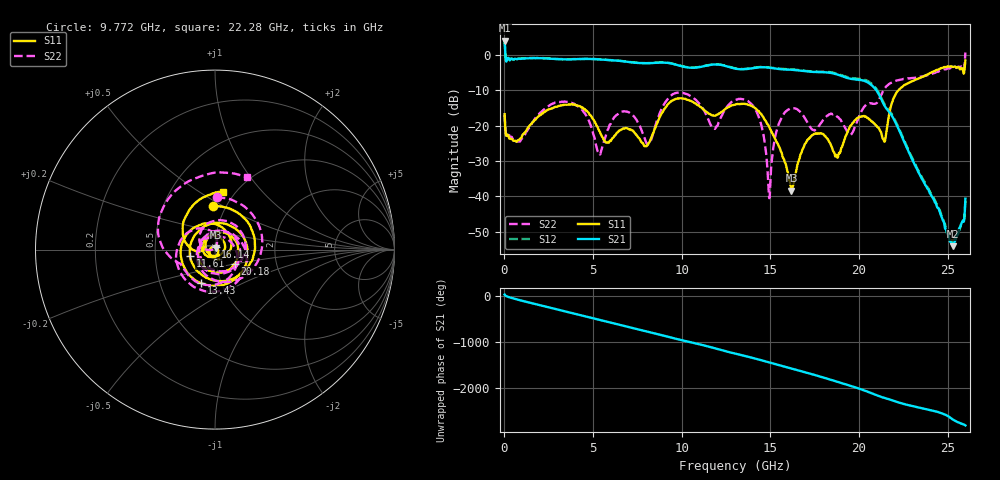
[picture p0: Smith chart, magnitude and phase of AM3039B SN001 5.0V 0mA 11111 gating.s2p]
!Agilent Technologies,E8364B,MY43040894,A.07.50.67
!Agilent E8364B: A.07.50.67
!Date: Tuesday, June 28, 2016 08:13:28
!Correction: S11(Full 2 Port(1,2))
!S21(Full 2 Port(1,2))
!S12(Full 2 Port(1,2))
!S22(Full 2 Port(1,2))
!S2P File: Measurements: S11, S21, S12, S22:
# Hz S  dB  R 50
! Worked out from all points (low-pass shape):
!   1601 points, 10 MHz to 26 GHz, reference 50 ohm
!   highest |S21| = 3.98 dB at 10 MHz (marker M1); lowest = -54.0 dB at 25.29 GHz (marker M2)
!   |S21| within 3 dB of the highest: start of sweep to 43.88 MHz
!   lowest |S11| = -38.3 dB at 16.19 GHz (marker M3), VSWR 1.02, Z = 50.6 + j1.06 ohm
!   |S11| at or under -10 dB: start of sweep to 22.22 GHz
!   |S22| runs from -40.5 to 0.6 dB; largest |S21 - S12| = 0.024
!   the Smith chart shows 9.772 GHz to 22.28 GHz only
!   S11 on the Smith chart (normalised r, x): 9.772 GHz: 0.87, +0.45; 11.61 GHz: 0.75, -0.06; 13.43 GHz: 0.80, -0.31; 16.14 GHz: 1.01, +0.03; 20.18 GHz: 1.23, -0.19; 22.28 GHz: 0.88, +0.64
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1e7  -16.77 53.1  3.98 41.1  4.04 41.9  -16.88 25.7
7.897e8  -24.12 22.4  -1.09 -75.0  -1.04 -74.9  -24.28 -12.7
1.813056e9  -17.89 -50.6  -0.92 -175.3  -0.88 -175.2  -17.44 -69.9
2.901388e9  -14.75 -175.7  -1.21 82.1  -1.15 82.2  -13.53 173.3
4.347081e9  -14.91 15.2  -1.20 -52.2  -1.17 -52.2  -15.43 11.1
5.549119e9  -23.37 -89.9  -1.40 -168.0  -1.35 -168.0  -25.61 -22.3
6.588719e9  -21.13 -131.2  -1.78 91.8  -1.75 92.0  -16.09 -109.6
8.684162e9  -18.48 -117.6  -2.24 -106.2  -2.19 -106.1  -17.58 -123.1
9.772494e9  -12.36 92.9  -2.97 144.8  -2.91 144.8  -10.71 88.2
1.160804e10  -16.82 -165.6  -2.88 -25.6  -2.83 -25.7  -19.49 -163.4
1.3005e10  -14.06 -56.2  -3.90 -168.8  -3.82 -168.6  -12.76 -78.4
1.342734e10  -13.87 -112.7  -4.11 152.0  -4.03 152.2  -12.54 -130.3
1.487303e10  -19.81 27.3  -3.63 4.1  -3.52 4.8  -35.53 78.5
1.614004e10  -37.01 77.6  -4.22 -128.8  -4.11 -128.2  -15.22 58.0
1.618878e10  -38.32 59.7  -4.24 -134.1  -4.14 -133.4  -15.08 51.2
1.734208e10  -22.79 168.9  -4.82 101.1  -4.71 101.9  -21.05 -160.0
1.891772e10  -27.79 -147.2  -5.80 -82.9  -5.59 -81.8  -18.14 -116.9
2.018474e10  -17.37 -35.0  -7.21 121.6  -6.89 123.0  -15.54 -55.5
2.167916e10  -17.40 177.1  -16.00 -85.9  -15.63 -85.5  -8.32 132.9
2.228018e10  -9.74 81.8  -21.55 -163.2  -21.13 -162.9  -7.10 65.8
2.528528e10  -3.44 146.1  -54.04 -167.8  -52.48 -161.2  -3.73 164.8
2.6e10  -1.60 47.8  -40.63 60.5  -40.48 62.7  0.63 76.5
